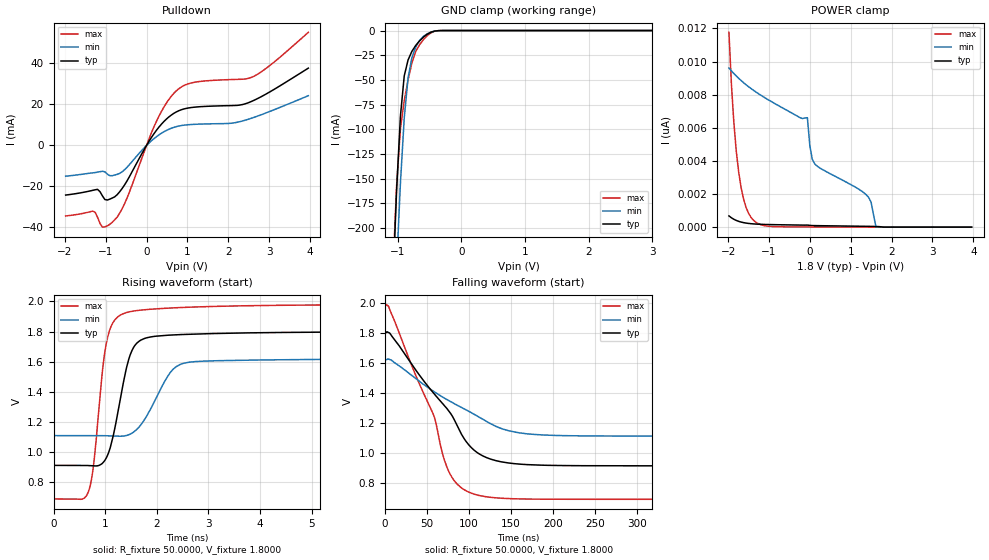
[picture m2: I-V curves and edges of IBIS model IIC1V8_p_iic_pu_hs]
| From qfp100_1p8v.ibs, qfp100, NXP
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[Model] IIC1V8_p_iic_pu_hs
|   Model IIC1V8_p_iic_pu_hs
| This model was characterised for following simulation conditions:
| External (pad) voltage:
|   - Typ: 1.8V,   - Min: 1.62V,   - Max: 1.98V
| Library cells for typ/min/max conditions are connected as defined below:
|  IO - External Pad
|  A - Core Input
|  EN - Output Buffer Enable
|  BOOST - vdde
|  ECS - vdd
|  EGP - gnd
|  ENZI - vdd
|  EPD - gnd
|  EPUN - vdd
|  SSEL - vdd
|  ZI - NC
|  ZIF - NC
|  gnd - gnd
|  gnde - gnde
|  vdd - vdd
|  vdde - vdde
| All other pins connected to ground
Model_type I/O_open_drain
Polarity   Non-Inverting
Enable   Active-Low
Vinl =   0.5400V
Vinh =   1.2600V
Vmeas =  0.9000V
Cref =   0.0F
Rref =   1000.000
Vref =   1.8000V
C_comp   3.6452pF   3.5037pF   3.7805pF
|C_comp_pullup   0.9521pF   0.9262pF   0.9623pF
|C_comp_pulldown   2.3411pF   2.4927pF   2.1971pF
[Model Spec]
| variable   typ   min   max
Vinh   0.5400V   0.4860V   0.5940V
Vinl   1.2600V   1.1340V   1.3860V
Vmeas   0.9000V   0.8100V   0.9900V
Vref   1.8000V   1.6200V   1.9800V
Cref   0.0F   0.0F   0.0F
Rref   1.0000k   1.0000k   1.0000k
[Temperature Range]   25.0000   0.1250k   -40.0000
[Voltage Range]   1.8000V   1.6200V   1.9800V
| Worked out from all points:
|   slope of the pulldown table from 0 to 0.27 V, typ, clamps not added: 33.4 ohm
|   GND clamp passes 1 mA (typ) near -0.44 V on its own axis
|   rising waveform, R_fixture 50.0000, V_fixture 1.8000: 20-80 % time 319ps typ, 487ps min, 235ps max; typ from 0.911 V to 1.8 V
|   falling waveform, R_fixture 50.0000, V_fixture 1.8000: 20-80 % time 66.9ns typ, 88.7ns min, 48.9ns max; typ from 1.8 V to 0.911 V
[Pulldown]
|Voltage   I(typ)   I(min)   I(max)
-1.98V    -24.22mA   -15.04mA   -34.42mA
-1.32V    -21.94mA   -13.4mA    -32.06mA
-1.2V     -21.45mA   -13.05mA   -35.06mA
-1.08V    -24.63mA   -12.6mA    -39.9mA
-900mV    -26.23mA   -14.78mA   -38.53mA
-720mV    -24.07mA   -14.13mA   -34.99mA
-540mV    -19.33mA   -11.9mA    -28.53mA
300mV     8.856mA    5.096mA    14.12mA
720mV     16.26mA    9.117mA    26.48mA
1.14V     18.6mA     10.26mA    30.69mA
2.58V     21.56mA    13.35mA    33.32mA
3.96V     37.73mA    24.28mA    55.2mA
[GND_clamp]
|Voltage   I(typ)   I(min)   I(max)
-1.98V    -2.104A    -2.075A    -2.136A
-1.08V    -259.3mA   -333mA     -246.9mA
-1.02V    -161.8mA   -238.7mA   -157.1mA
-960mV    -86.74mA   -154.7mA   -99.46mA
-900mV    -45.95mA   -88.82mA   -71.05mA
-840mV    -29.9mA    -47.99mA   -50.25mA
-780mV    -21.15mA   -27.64mA   -32.98mA
-720mV    -15.16mA   -16.87mA   -21.26mA
-660mV    -10.56mA   -10.24mA   -14.56mA
-540mV    -3.788mA   -3.398mA   -5.292mA
-300mV    -15.94uA   -36uA      -16.34uA
3.96V     0A         0A         0A
[POWER_clamp]
|Voltage   I(typ)   I(min)   I(max)
-1.98V    679.6pA    9.61nA     11.76nA
-1.86V    475.2pA    9.277nA    6.313nA
-1.74V    349.2pA    8.982nA    3.292nA
-1.56V    245.6pA    8.597nA    1.186nA
-1.32V    186pA      8.161nA    293.2pA
-60mV     124.8pA    6.606nA    14.31pA
0V        105.5pA    4.916nA    11.81pA
120mV     93.21pA    3.82nA     10.91pA
1.38V     50pA       1.96nA     2.877pA
1.5V      45.28pA    1.501nA    2.149pA
1.62V     39.18pA    0A         1.42pA
3.96V     0A         0A         0A
[Ramp]
| variable   typ   min   max
dV/dt_r  0.5334/0.3186n   0.3066/0.4865n   0.7753/0.2353n
dV/dt_f  0.5334/66.9335n   0.3066/88.7039n   0.7753/48.9313n
R_load = 50.0000
[Rising Waveform]
R_fixture= 50.0000
V_fixture= 1.8000
V_fixture_min= 1.6200
V_fixture_max= 1.9800
|time   V(typ)   V(min)   V(max)
0s        911mV      1.109V     687.8mV
674.7ps   909.7mV    1.109V     735mV
774ps     907.3mV    1.109V     907.6mV
1.008ns   951.7mV    1.108V     1.695V
1.271ns   1.308V     1.105V     1.904V
1.478ns   1.639V     1.117V     1.932V
1.767ns   1.755V     1.217V     1.945V
2.535ns   1.781V     1.591V     1.961V
5.708ns   1.797V     1.616V     1.978V
1us       1.8V       1.62V      1.98V
[Falling Waveform]
R_fixture= 50.0000
V_fixture= 1.8000
V_fixture_min= 1.6200
V_fixture_max= 1.9800
|time   V(typ)   V(min)   V(max)
0s        1.8V       1.62V      1.98V
4.113ns   1.8V       1.623V     1.974V
57.98ns   1.394V     1.407V     1.245V
67.73ns   1.331V     1.373V     1.005V
75.59ns   1.279V     1.347V     875.9mV
89.4ns    1.138V     1.305V     770.9mV
112.2ns   990.4mV    1.235V     713.1mV
146.9ns   930.5mV    1.146V     692.8mV
205.4ns   913.7mV    1.114V     688.4mV
1us       911.1mV    1.109V     687.9mV
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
